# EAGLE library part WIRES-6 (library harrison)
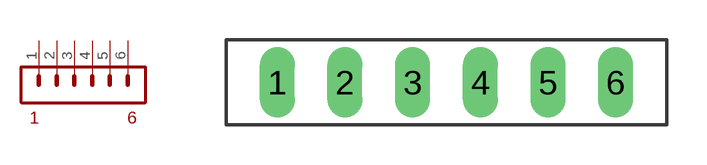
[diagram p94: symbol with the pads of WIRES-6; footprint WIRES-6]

Designator prefix S

## WIRES-6  [WIRES-6]
1  1  pas
2  2  pas
3  3  pas
4  4  pas
5  5  pas
6  6  pas

## Footprint WIRES-6 (pad centres in mm)
drill 0.813 long: 1 -6.35,0; 2 -3.81,0; 3 -1.27,0; 4 1.27,0; 5 3.81,0; 6 6.35,0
